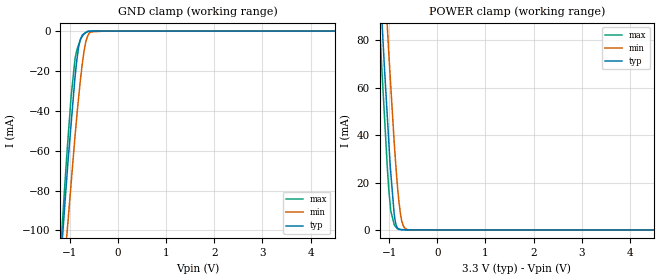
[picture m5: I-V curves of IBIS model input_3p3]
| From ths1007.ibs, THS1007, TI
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|   input_3p3 Model
[Model]   input_3p3
Model_type   Input
Vinl = 0.6
Vinh = 2
|   typ   min   max
|   (nom PVT)   (fast PVT)   (slow PVT)
C_comp   1.043e-12   1.039e-12   1.060e-12
| Where nom  PVT is Nominal Process, 3.3V, 27C
| Fast PVT is Strong Process,  3.6V, -40C
| Slow PVT is Weak Process,   3V, 125C
[Voltage Range]   3.3   3   3.6
|Ambient Temperature   25   85   -40
|Junction Temperature
[Temperature Range]   27   125   -40
[Power Clamp Reference]   3.3   3   3.6
[GND Clamp Reference]   0   0   0
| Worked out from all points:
|   GND clamp passes 1 mA (typ) near -0.68 V on its own axis
|   POWER clamp passes 1 mA (typ) near -0.83 V on its own axis
[GND Clamp]
|   Voltage   I(typ)   I(min)   I(max)
-3.3V     -955.2mA   -917.9mA   -1.014A
-1.224V   -126.5mA   -152.6mA   -120.7mA
-1.109V   -86.98mA   -115.8mA   -77.04mA
-1.062V   -71.76mA   -101mA     -60.28mA
-979.2mV  -46.88mA   -76.77mA   -33.12mA
-896.4mV  -22.99mA   -52.58mA   -13.93mA
-821.7mV  -8.072mA   -33.28mA   -6.791mA
-785.4mV  -4.157mA   -24.71mA   -4.431mA
-714mV    -1.471mA   -10.82mA   -1.615mA
-633.6mV  -182.5uA   -2.478mA   -195.1uA
-285mV    -13.98uA   -318nA     -92.94nA
6.6V      0A         0A         0A
[POWER Clamp]
|   Voltage   I(typ)   I(min)   I(max)
-3.3V     1.011A     1.029A     1.01A
-1.284V   140.1mA    178.9mA    120.5mA
-1.155V   89.3mA     128.4mA    68.2mA
-1.099V   68.06mA    107.6mA    47.73mA
-1.037V   46.57mA    84.52mA    25.23mA
-968.4mV  24.15mA    60.66mA    8.003mA
-897.6mV  6.761mA    37.1mA     2.296mA
-810mV    492.5uA    14.23mA    237.7uA
-765mV    191.7uA    6.561mA    184.2uA
-714mV    66.85uA    2.047mA    123.5uA
-591mV    55.28uA    69.38uA    15.7uA
6.6V      0A         0A         0A
